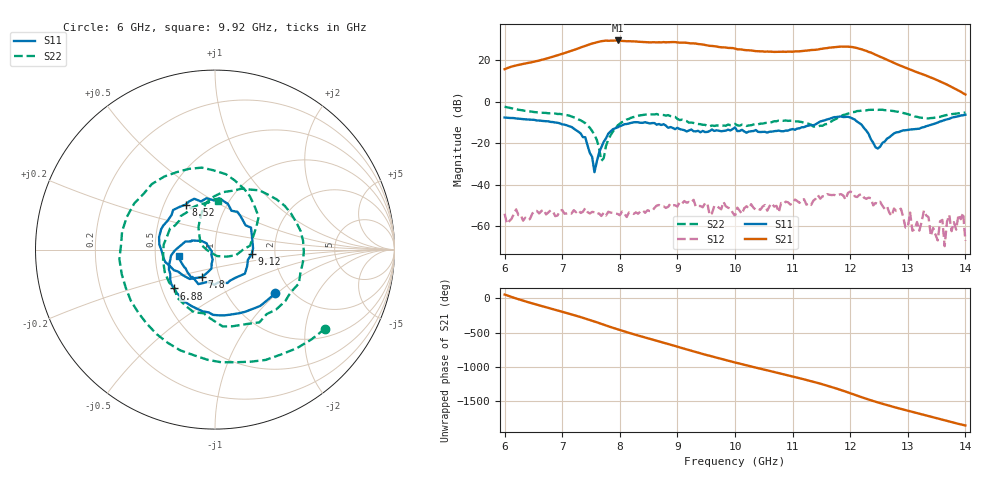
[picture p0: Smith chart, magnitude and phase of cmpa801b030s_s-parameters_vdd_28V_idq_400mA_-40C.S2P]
!Keysight Technologies,E5071C,MY46110325,B.14.03
!Date: Tue Aug 11 10:39:29 2020
!Data & Calibration Information:
!Freq	S11:SOLT2(ON)	S21:SOLT2(ON)	S12:SOLT2(ON)	S22:SOLT2(ON)
!PortZ  Port1:50+j0  Port2:50+j0
!Above PortZ is port z conversion or system Z0 setting when saving the data.
!When reading, reference impedance value at option line is always used.
# Hz S dB R 50
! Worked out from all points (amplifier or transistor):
!   201 points, 6 GHz to 14 GHz, reference 50 ohm
!   highest |S21| = 29.5 dB at 7.96 GHz (marker M1)
!   |S21| within 3 dB of that: 7.362 GHz to 9.696 GHz (2.335 GHz wide, 27.4 % of centre)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
!   unconditionally stable (mu >= 1): start of sweep to end of sweep
!   at 7.32 GHz: K = 10.13, MAG = 26.8 dB, |S12| = -53.6 dB
!   at 10 GHz: K = 12.97, MAG = 26.2 dB, |S12| = -55.1 dB
!   at 14 GHz: K = 406.00, MAG = 6.2 dB, |S12| = -67.1 dB
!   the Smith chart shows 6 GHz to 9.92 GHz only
!   S11 on the Smith chart (normalised r, x): 6 GHz: 1.65, -0.97; 6.88 GHz: 0.58, -0.28; 7.8 GHz: 0.83, -0.26; 8.52 GHz: 0.64, +0.35; 9.12 GHz: 1.51, -0.08; 9.92 GHz: 0.67, -0.05
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6e9  -7.65 -36.1  15.67 56.1  -54.00 174.7  -2.44 -35.7
6.88e9  -10.05 -136.5  22.05 -167.0  -55.19 24.9  -5.71 150.3
7.36e9  -17.09 160.9  26.49 75.9  -53.07 -67.5  -9.64 48.5
7.64e9  -24.63 -102.8  28.90 -1.1  -53.87 -137.2  -22.40 -31.1
7.8e9  -15.40 -115.2  29.35 -48.1  -53.03 178.7  -18.28 136.0
7.96e9  -12.42 -149.2  29.51 -92.5  -54.08 106.6  -11.55 101.1
8.24e9  -9.92 167.5  29.07 -163.9  -54.09 34.9  -7.41 45.8
8.52e9  -10.47 123.2  28.59 129.1  -52.72 -40.2  -6.11 -1.2
8.68e9  -10.75 99.4  28.64 90.7  -49.78 -75.1  -6.30 -29.6
9.12e9  -13.75 -7.4  28.45 -15.3  -47.88 -176.6  -9.00 -116.8
9.44e9  -14.12 -91.3  27.55 -93.0  -50.91 114.9  -11.14 165.0
9.92e9  -13.87 -169.5  25.85 161.1  -51.53 -4.8  -11.33 86.5
1e10  -12.39 172.2  25.60 142.2  -55.12 -37.3  -10.70 75.1
1.068e10  -14.21 77.7  23.99 3.6  -50.59 -158.6  -9.41 -30.7
1.104e10  -13.56 44.0  24.25 -70.8  -47.17 139.0  -9.50 -83.1
1.136e10  -11.39 15.9  24.93 -140.4  -47.73 94.3  -11.97 -154.2
1.164e10  -8.27 -12.0  26.03 153.5  -44.87 13.5  -9.98 114.0
1.188e10  -7.41 -44.8  26.54 88.1  -45.24 -58.5  -6.40 38.3
1.216e10  -10.34 -95.2  25.49 6.2  -44.91 -138.1  -4.47 -42.1
1.24e10  -19.83 -169.8  23.13 -60.7  -50.01 144.3  -3.92 -101.3
1.268e10  -17.15 55.8  19.64 -130.6  -53.55 82.1  -4.27 -153.6
1.4e10  -6.29 -164.7  3.47 -58.3  -67.09 -59.2  -5.23 -43.0
